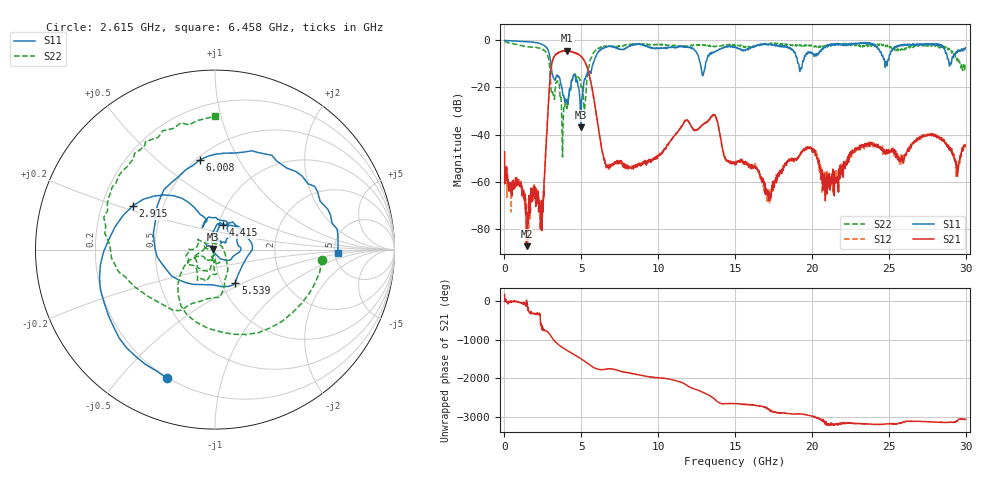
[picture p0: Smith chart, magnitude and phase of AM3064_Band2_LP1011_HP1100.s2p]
# Hz S DB R 50.0
!freq dBS11 angS11 dBS21 angS21 dBS12 angS12 dBS22 angS22
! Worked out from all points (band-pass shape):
!   1600 points, 10 MHz to 29.98 GHz, reference 50 ohm
!   highest |S21| = -4.33 dB at 4.059 GHz (marker M1); lowest = -87.5 dB at 1.435 GHz (marker M2)
!   |S21| within 3 dB of the highest: 3.2 GHz to 5.057 GHz (1.857 GHz wide, 45 % of centre)
!   lowest |S11| = -36.9 dB at 4.977 GHz (marker M3), VSWR 1.03, Z = 48.7 + j0.394 ohm
!   |S11| at or under -10 dB: 3.021 GHz to 5.755 GHz (2.734 GHz wide, 62.3 % of centre); 12.75 GHz to 13.08 GHz (335.1 MHz wide, 2.6 % of centre); 19.14 GHz to 19.37 GHz (238.1 MHz wide, 1.24 % of centre)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
!   |S22| runs from -49.5 to -0.3 dB; largest |S21 - S12| = 0.02
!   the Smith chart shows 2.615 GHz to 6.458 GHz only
!   S11 on the Smith chart (normalised r, x): 2.615 GHz: 0.20, -0.68; 2.915 GHz: 0.34, +0.22; 4.415 GHz: 1.05, +0.29; 5.539 GHz: 1.16, -0.45; 6.008 GHz: 0.52, +0.70; 6.458 GHz: 5.31, -0.34
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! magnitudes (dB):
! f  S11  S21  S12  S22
! 10 MHz  0.0  -47.3  -57.5  -0.3
! 1.435 GHz  -0.5  -87.5  -69.1  -2.6
! 2.372 GHz  -1.5  -75.2  -69.3  -3.5
! 2.615 GHz  -2.3  -56.3  -55.5  -4.4
! 2.915 GHz  -5.7  -20.7  -20.7  -9.8
! 3.215 GHz  -16.3  -7.2  -7.1  -24.8
! 4.059 GHz  -26.1  -4.3  -4.5  -29.0
! 4.415 GHz  -16.8  -5.0  -4.8  -16.9
! 4.977 GHz  -36.9  -6.8  -6.8  -18.9
! 5.015 GHz  -25.9  -7.0  -7.0  -20.1
! 5.539 GHz  -13.3  -15.3  -15.1  -9.8
! 6.008 GHz  -5.9  -32.8  -32.8  -3.7
! 6.458 GHz  -3.3  -50.2  -50.0  -2.6
! 10 GHz  -3.4  -48.7  -49.0  -1.9
! 12.91 GHz  -15.0  -35.8  -35.7  -2.0
! 13.6 GHz  -4.9  -31.8  -31.8  -2.5
! 15 GHz  -2.7  -53.0  -52.2  -1.9
! 17.18 GHz  -2.0  -68.0  -67.9  -1.6
! 19.99 GHz  -5.2  -46.1  -45.9  -2.0
! 20.85 GHz  -2.9  -59.1  -58.2  -2.6
! 25 GHz  -8.1  -47.3  -47.4  -2.2
! 29.98 GHz  -3.1  -44.6  -45.4  -10.3
